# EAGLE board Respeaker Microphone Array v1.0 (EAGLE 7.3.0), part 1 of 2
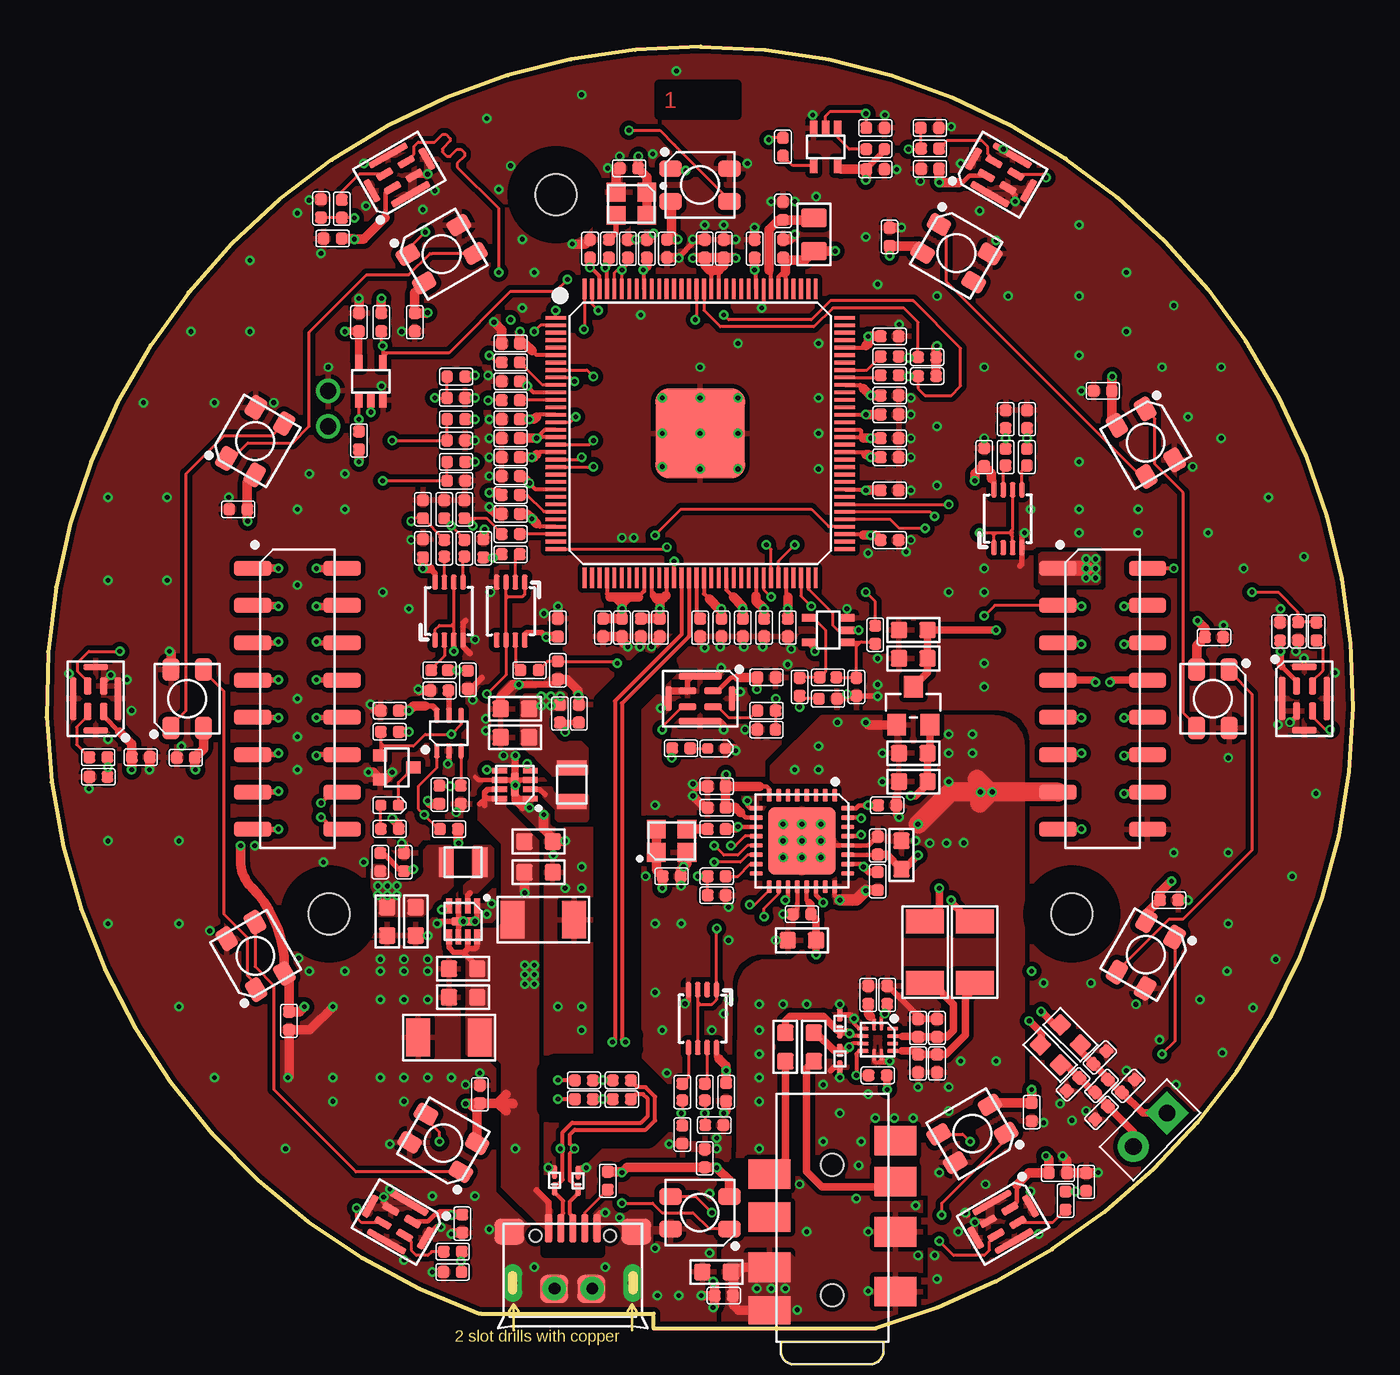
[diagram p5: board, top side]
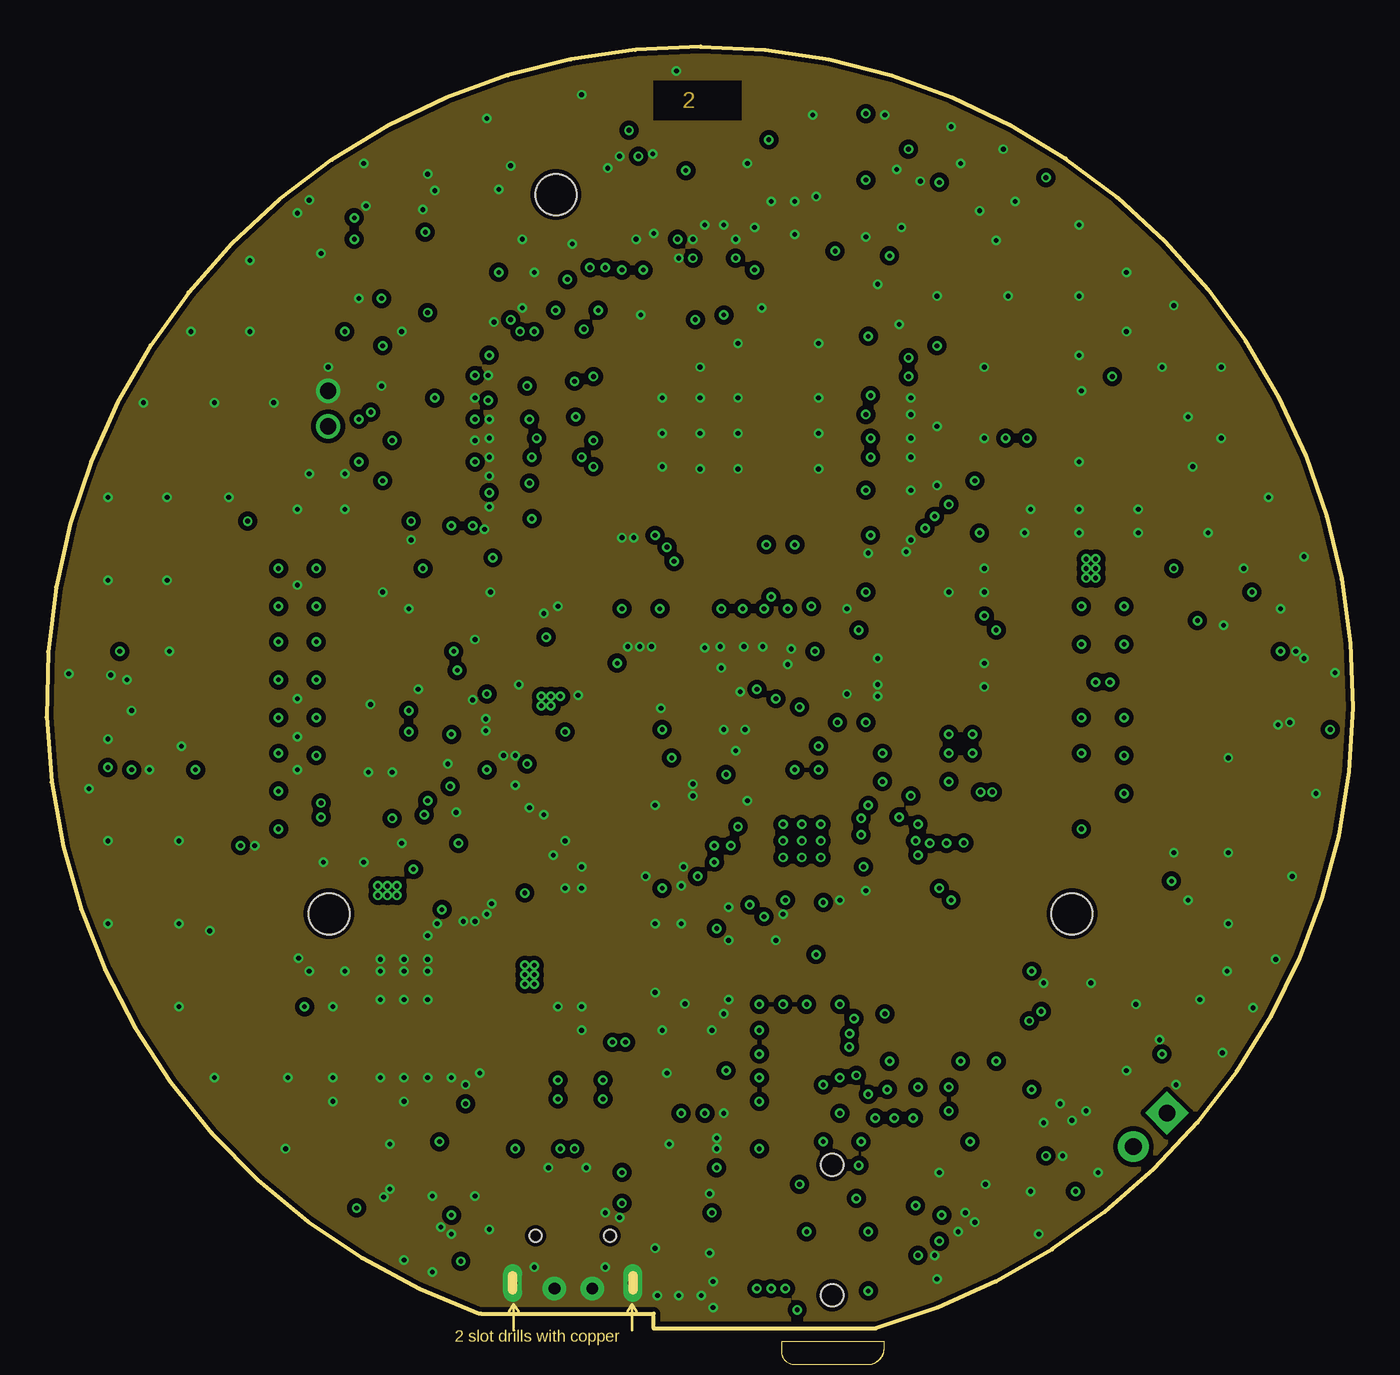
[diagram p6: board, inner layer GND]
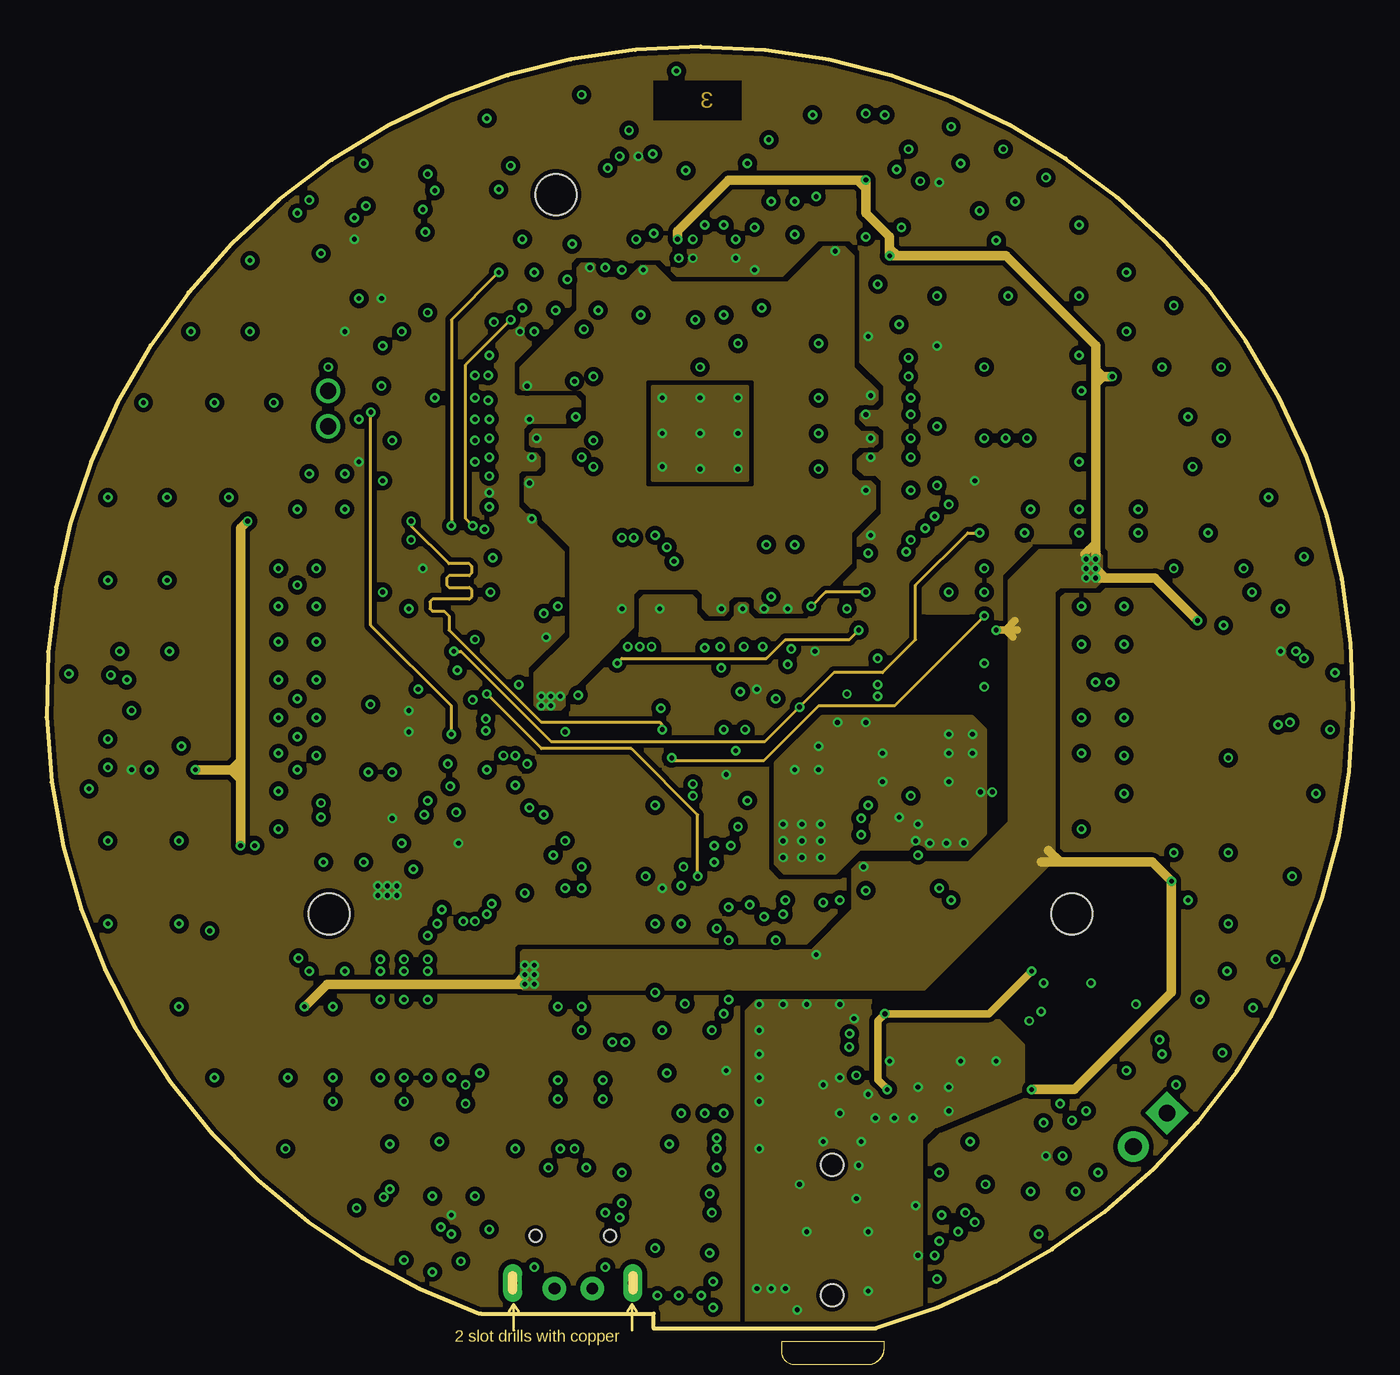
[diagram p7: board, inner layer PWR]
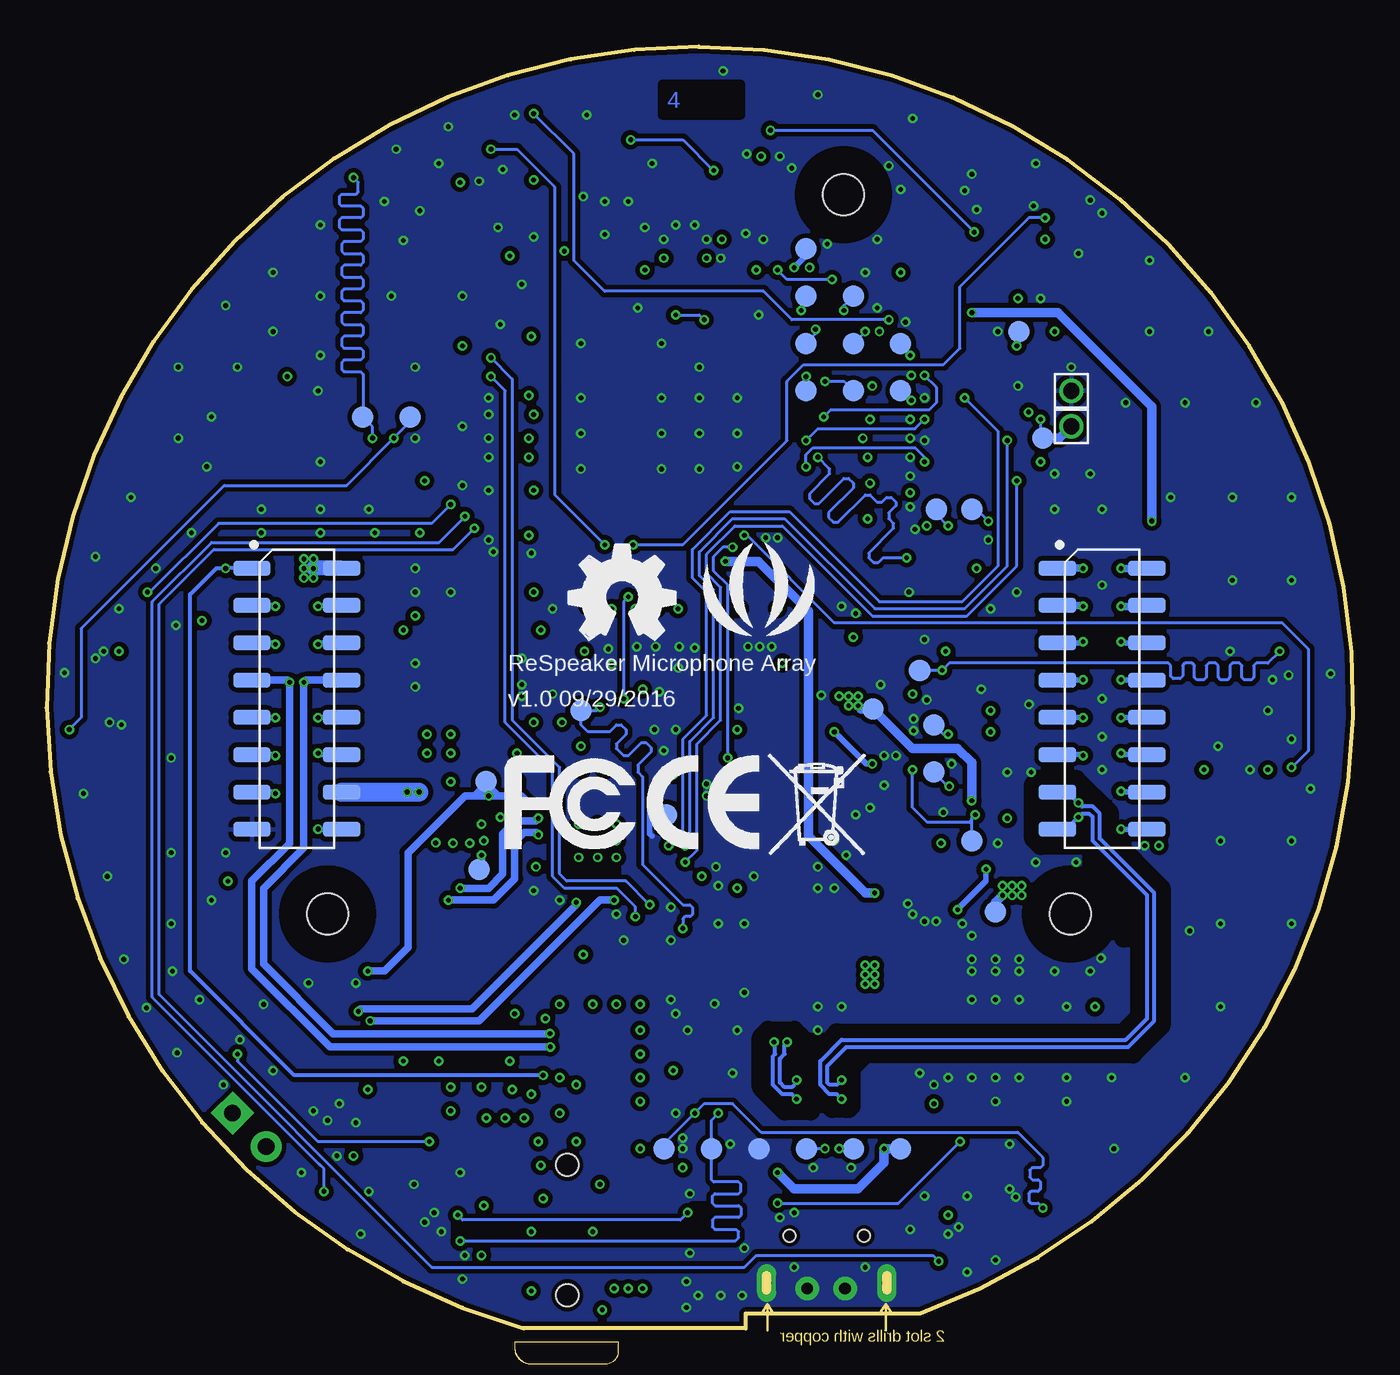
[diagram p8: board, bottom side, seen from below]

Size 70.04 x 68.72 mm. Coordinates in mm from the lower left corner, seen from the top.
Outline: 32.55,0 44.46,0
Outline: 23.28,0.79 32.55,0.79 32.55,0.03
Outline: 35.06,68.72 arc-164 44.47,0.01
Outline: 35.06,68.71 arc161 23.23,0.79
Copper layers (1*2*15*16): Top 0.035mm / dielectric 0.2mm / GND 0.0175mm / dielectric 0.3mm / PWR 0.0175mm / dielectric 0.2mm / Bottom 0.035mm
Design rules "SeeedStudio_4layer_DRU_no_angle_20140221 *": minimum track width 1mil, minimum drill 8mil, track to track 6mil, track to pad 6mil, pad to pad 6mil, via to via 6mil, smd to smd 0mil, copper to edge 10mil, drill to drill 8mil, minimum pad ring 6mil, minimum via ring 4mil, stop-mask expansion 4mil, vias tented up to drill 25mil, thermal gap 10mil
Net classes: 0 default: width 0.025 mm, drill 0.203 mm, clearance 0.102 mm
Holes 2.2 mm at 15.14,22.22 54.98,22.22 27.3,60.78
tRestrict: area 22.1,24.2 to 22.5,25.8; area 27.4,28.9 to 28.9,29.4; area 52.6,19.9 to 57.3,24.6; area 12.8,19.9 to 17.5,24.6; area 25,58.4 to 29.7,63.1; area 32.8,65 to 37,66.7; area 36.8,8.2 to 37.3,8.9; area 48.2,10.2 to 50.3,11.9; area 34.9,25.2 to 35.4,25.8; 19 lines
bRestrict: area 52.6,19.9 to 57.3,24.6; area 12.8,19.9 to 17.5,24.6; area 25,58.4 to 29.7,63.1; area 32.8,65 to 37,66.7; area 39.5,24.2 to 41.8,24.9; area 35.5,5.1 to 48.1,5.6; area 34.7,6.1 to 35.4,6.6; 33 lines

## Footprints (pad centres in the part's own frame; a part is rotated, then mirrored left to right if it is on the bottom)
TP-D45MIL = smd 1.143 x 1.143: T 0,0
C0402 = smd 0.635 x 0.635: 1 0,0.484; 2 0,-0.484
C0603 = smd 0.889 x 0.889: 1 0,0.762; 2 0,-0.762
C1206 = smd 1.27 x 2.032: 1 -1.651,0; 2 1.651,0
SOD-923 = smd 0.7 x 0.3: 1 -0.45,0; 2 0.45,0
LED-0402 = smd 0.58 x 0.58: + -0.468,0; - 0.468,0
MICRO-USB5+4P-SMD-0.65-B = smd 0.381 x 1.524: 1 -1.3,-0.25; 2 -0.65,-0.25; 3 0,-0.25; 4 0.65,-0.25; 5 1.3,-0.25 | smd 1.6 x 1.397: S1 -3.4,-0.427; S6 3.4,-0.427 | drill 0.508 pad 1.016 long: S2 -3.226,-3.175; S5 3.226,-3.175 | smd 1.5 x 1.5: S3 -1,-3.5; S4 1,-3.5 | hole 0.635: -2,-0.65; 2,-0.65
H2X8-SMD-2.0 = smd 2 x 0.8: 1 -2.4,7; 2 2.4,7; 3 -2.4,5; 4 2.4,5; 5 -2.4,3; 6 2.4,3; 7 -2.4,1; 8 2.4,1; 9 -2.4,-1; 10 2.4,-1; 11 -2.4,-3; 12 2.4,-3; 13 -2.4,-5; 14 2.4,-5; 15 -2.4,-7; 16 2.4,-7
1P-40/25MIL = drill 0.864 pad 1.27: 1 0,0
AUDIO8P-SMD-3.5-14.5X6.1X4.0MM = smd 1.6 x 2.25: 1 3.9,-3.375; 2 7.1,-3.375; 3 9.8,-3.375; 4 10.2,3.375; 6 5.2,3.375; 7 7.9,3.375; 8 12,-3.375 | smd 1.5 x 2.25: 5 2.9,3.375 | hole 1.2: 3.7,0; 10.7,0
H2-2.54 = drill 0.889 pad 1.651 square: 1 0,1.27 | drill 0.889 pad 1.651: 2 0,-1.27
L201610 = smd 0.8 x 1.6: 1 -0.9,0; 2 0.9,0
L0603 = smd 0.889 x 0.889: 1 -0.762,0; 2 0.762,0
HCLGA5P-3X4X1MM = smd 0.95 x 0.4: 1 -0.675,-0.425; 2 0.675,-0.425; 3 0.675,0.425; 4 -0.675,0.425 | smd 2.3 x 0.35: 5 0,-1.2; 7 0,1.2 | smd 0.35 x 1.3: 6 1.7,0; 8 -1.7,0
SOT-323 = smd 0.635 x 0.762: 1 -0.635,-0.889; 2 0.635,-0.889; 3 0,0.889
R0402 = smd 0.635 x 0.635: 1 0,0.484; 2 0,-0.484
R0805 = smd 1.397 x 1.016: 1 0,0.889; 2 0,-0.889
R0402' = smd 0.635 x 0.635: 1 0,0.445; 2 0,-0.445
LED4-SMD-3.5X3.7MM = smd 1.2 x 0.9: 1 -1.58,0.875; 2 -1.58,-0.875; 3 1.58,-0.875; 4 1.58,0.875
LEAD12P-SMD-0.4-1.8X1.8X0.5MM = smd 0.6 x 0.2: 1 -0.8,0.2; 2 -0.8,-0.2; 7 0.8,-0.2; 8 0.8,0.2 | smd 0.2 x 0.6: 3 -0.6,-0.8; 4 -0.2,-0.8; 5 0.2,-0.8; 6 0.6,-0.8; 9 0.6,0.8; 10 0.2,0.8; 11 -0.2,0.8; 12 -0.6,0.8
TQFP128-0.4-14X14MM = smd 1.1 x 0.2: 1 -7.75,6.2; 2 -7.75,5.8; 3 -7.75,5.4; 4 -7.75,5; 5 -7.75,4.6; 6 -7.75,4.2; 7 -7.75,3.8; 8 -7.75,3.4; 9 -7.75,3; 10 -7.75,2.6; 11 -7.75,2.2; 12 -7.75,1.8; 13 -7.75,1.4; 14 -7.75,1; 15 -7.75,0.6; 16 -7.75,0.2; 17 -7.75,-0.2; 18 -7.75,-0.6; 19 -7.75,-1; 20 -7.75,-1.4; 21 -7.75,-1.8; 22 -7.75,-2.2; 23 -7.75,-2.6; 24 -7.75,-3; 25 -7.75,-3.4; 26 -7.75,-3.8; 27 -7.75,-4.2; 28 -7.75,-4.6; 29 -7.75,-5; 30 -7.75,-5.4; 31 -7.75,-5.8; 32 -7.75,-6.2; 65 7.75,-6.2; 66 7.75,-5.8; 67 7.75,-5.4; 68 7.75,-5; 69 7.75,-4.6; 70 7.75,-4.2; 71 7.75,-3.8; 72 7.75,-3.4; 73 7.75,-3; 74 7.75,-2.6; 75 7.75,-2.2; 76 7.75,-1.8; 77 7.75,-1.4; 78 7.75,-1; 79 7.75,-0.6; 80 7.75,-0.2; 81 7.75,0.2; 82 7.75,0.6; 83 7.75,1; 84 7.75,1.4; 85 7.75,1.8; 86 7.75,2.2; 87 7.75,2.6; 88 7.75,3; 89 7.75,3.4; 90 7.75,3.8; 91 7.75,4.2; 92 7.75,4.6; 93 7.75,5; 94 7.75,5.4; 95 7.75,5.8; 96 7.75,6.2 | smd 0.2 x 1.1: 33 -6.2,-7.75; 34 -5.8,-7.75; 35 -5.4,-7.75; 36 -5,-7.75; 37 -4.6,-7.75; 38 -4.2,-7.75; 39 -3.8,-7.75; 40 -3.4,-7.75; 41 -3,-7.75; 42 -2.6,-7.75; 43 -2.2,-7.75; 44 -1.8,-7.75; 45 -1.4,-7.75; 46 -1,-7.75; 47 -0.6,-7.75; 48 -0.2,-7.75; 49 0.2,-7.75; 50 0.6,-7.75; 51 1,-7.75; 52 1.4,-7.75; 53 1.8,-7.75; 54 2.2,-7.75; 55 2.6,-7.75; 56 3,-7.75; 57 3.4,-7.75; 58 3.8,-7.75; 59 4.2,-7.75; 60 4.6,-7.75; 61 5,-7.75; 62 5.4,-7.75; 63 5.8,-7.75; 64 6.2,-7.75; 97 6.2,7.75; 98 5.8,7.75; 99 5.4,7.75; 100 5,7.75; 101 4.6,7.75; 102 4.2,7.75; 103 3.8,7.75; 104 3.4,7.75; 105 3,7.75; 106 2.6,7.75; 107 2.2,7.75; 108 1.8,7.75; 109 1.4,7.75; 110 1,7.75; 111 0.6,7.75; 112 0.2,7.75; 113 -0.2,7.75; 114 -0.6,7.75; 115 -1,7.75; 116 -1.4,7.75; 117 -1.8,7.75; 118 -2.2,7.75; 119 -2.6,7.75; 120 -3,7.75; 121 -3.4,7.75; 122 -3.8,7.75; 123 -4.2,7.75; 124 -4.6,7.75; 125 -5,7.75; 126 -5.4,7.75; 127 -5.8,7.75; 128 -6.2,7.75 | smd 4.8 x 4.8: PAD 0,0
DFN8G-0.5-2X2MM = smd 0.8 x 0.3: 1 -0.827,0.75; 2 -0.827,0.25; 3 -0.827,-0.25; 4 -0.827,-0.75; 5 0.827,-0.75; 6 0.827,-0.25; 7 0.827,0.25; 8 0.827,0.75 | smd 0.45 x 1.3: 9 0,0
SOT-353 = smd 0.4 x 0.8: 1 -0.65,-1; 2 0,-1; 3 0.65,-1; 4 0.65,1; 5 -0.65,1
SC-70-6 = smd 0.3 x 0.8: 1 -0.65,-0.95; 2 0,-0.95; 3 0.65,-0.95; 4 0.65,0.95; 5 0,0.95; 6 -0.65,0.95
QFN32G-0.5-5X5MM = smd 0.7 x 0.25: 1 -2.45,1.75; 2 -2.45,1.25; 3 -2.45,0.75; 4 -2.45,0.25; 5 -2.45,-0.25; 6 -2.45,-0.75; 7 -2.45,-1.25; 8 -2.45,-1.75; 17 2.45,-1.75; 18 2.45,-1.25; 19 2.45,-0.75; 20 2.45,-0.25; 21 2.45,0.25; 22 2.45,0.75; 23 2.45,1.25; 24 2.45,1.75 | smd 0.25 x 0.7: 9 -1.75,-2.45; 10 -1.25,-2.45; 11 -0.75,-2.45; 12 -0.25,-2.45; 13 0.25,-2.45; 14 0.75,-2.45; 15 1.25,-2.45; 16 1.75,-2.45; 25 1.75,2.45; 26 1.25,2.45; 27 0.75,2.45; 28 0.25,2.45; 29 -0.25,2.45; 30 -0.75,2.45; 31 -1.25,2.45; 32 -1.75,2.45 | smd 3.6 x 3.6: 33 0,0
SOT-23 = smd 1.016 x 1.143: 1 -0.889,-1.016; 2 0.889,-1.016; 3 0,1.016
US-8 = smd 0.8 x 0.3: 1 -1.55,0.75; 2 -1.55,0.25; 3 -1.55,-0.25; 4 -1.55,-0.75; 5 1.55,-0.75; 6 1.55,-0.25; 7 1.55,0.25; 8 1.55,0.75
OSC-SMD-2.5X2.0X0.9MM = smd 1 x 1: 1 -0.825,-0.625; 2 0.825,-0.625; 3 0.825,0.625; 4 -0.825,0.625

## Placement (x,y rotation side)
1V  [TP-D45MIL]  25.74,33.21 90 bottom
3V3  [TP-D45MIL]  19.17,22.34 180 bottom
24M  [TP-D45MIL]  29.33,57.89 270 bottom
24M_1  [TP-D45MIL]  36.81,27.53 0 bottom
ADM_VIN  [TP-D45MIL]  22.46,29.82 270 bottom
C1  100nF  [C0402]  36.43,12.67 180 top
C2  100nF  [C0402]  33.51,24.23 270 top
C3  10uF  [C0603]  46.47,37.44 90 top
C4  100nF  [C0402]  44.56,25.88 0 top
C5  100nF  [C0402]  27.41,37.57 0 top
C6  10uF  [C0603]  22.33,19.28 90 top
C7  10uF  [C0603]  22.33,17.75 90 top
C8  10uF  [C0603]  18.27,21.82 180 top
C9  10uF  [C0603]  19.79,21.82 180 top
C10  100uF 10V  [C1206]  21.57,15.6 0 top
C11  100nF  [C0402]  19.73,53.95 180 top
C12  100nF  [C0402]  10.27,43.91 90 top
C13  100nF  [C0402]  7.46,30.6 90 top
C14  100nF  [C0402]  13,16.49 180 top
C15  100nF  [C0402]  23.23,12.55 0 top
C16  100nF  [C0402]  35.29,9.12 0 top
C17  10uF  [C0603]  46.47,35.92 90 top
C18  10uF  [C0603]  25.11,31.69 90 top
C19  10uF  [C0603]  26.38,26.1 270 top
C20  10uF  [C0603]  25.11,33.21 90 top
C21  10uF  [C0603]  26.38,24.45 270 top
C22  100uF 10V  [C1206]  26.63,21.91 180 top
C23  100nF  [C0402]  39.48,59.91 0 top
C24  100nF  [C0402]  31.23,62.2 90 top
C25  100nF  [C0402]  45.2,44.93 270 top
C26  100nF  [C0402]  32.18,57.89 0 top
C27  100nF  [C0402]  45.2,50.01 270 top
C28  100nF  [C0402]  24.88,47.73 90 top
C29  100nF  [C0402]  24.88,50.77 90 top
C30  100nF  [C0402]  45.2,47.73 270 top
C31  100nF  [C0402]  39.49,57.89 0 top
C32  100nF  [C0402]  29.14,57.89 0 top
C33  100nF  [C0402]  24.88,45.69 90 top
C34  100nF  [C0402]  29.83,37.57 180 top
C35  100nF  [C0402]  30.85,37.57 180 top
C36  100nF  [C0402]  36.18,37.57 180 top
C37  100nF  [C0402]  38.47,37.57 180 top
C38  100nF  [C0402]  39.74,37.57 180 top
C39  100nF  [C0402]  35.3,57.89 0 top
C40  100nF  [C0402]  24.88,43.66 90 top
C41  100nF  [C0402]  32.88,37.57 180 top
C42  100nF  [C0402]  31.87,37.57 180 top
C43  100nF  [C0402]  24.88,46.71 90 top
C44  100nF  [C0402]  24.88,48.74 90 top
C45  100nF  [C0402]  24.88,52.81 90 top
C46  100nF  [C0402]  37.33,37.57 180 top
C47  100nF  [C0402]  45.2,42.27 270 top
C48  100nF  [C0402]  45.2,46.71 270 top
C49  100nF  [C0402]  45.2,49 270 top
C50  100nF  [C0402]  45.2,53.19 270 top
C51  100nF  [C0402]  37.96,57.89 0 top
C52  100nF  [C0402]  36.31,57.89 0 top
C53  100nF  [C0402]  52.82,11.6 180 top
C54  100nF  [C0402]  60.18,22.97 270 top
C55  100nF  [C0402]  38.6,34.9 270 top
C56  100nF  [C0402]  15.33,58.43 90 top
C57  100nF  [C0402]  5.05,30.63 270 top
C58  100nF  [C0402]  22.28,5.62 180 top
C59  100nF  [C0402]  54.22,8.33 270 top
C60  100nF  [C0402]  66.13,37.36 0 top
C61  100nF  [C0402]  47.37,62.17 90 top
C62  100nF  [C0402]  44.56,23.98 180 top
C63  2.2nF  [C0402]  21.06,34.2 90 top
C64  100nF  [C0402]  18.4,33.12 90 top
C65  100nF  [C0402]  16.74,53.95 0 top
C66  100nF  [C0402]  31.17,57.89 0 top
C67  100nF  [C0402]  50.27,46.71 0 top
C68  10uF  [C0603]  46.47,30.84 90 top
C69  100nF  [C0402]  40.5,22.2 90 top
C70  100nF  [C0402]  20.18,41.82 0 top
C71  10uF  [C0603]  46.47,29.31 90 top
C72  100nF  [C0402]  62.59,37.06 270 top
C73  100nF  [C0402]  56.63,50.26 90 top
C74  100nF  [C0402]  45.19,58.52 0 top
C75  100nF  [C0402]  33.26,57.89 180 top
C76  100nF  [C0402]  44.43,62.14 270 top
C77  1.5nF  [C0402]  22.4,43.92 180 top
C78  100pF  [C0402]  35.92,23.22 270 top
C79  100nF  [C0402]  45.07,17.88 0 top
C80  1.5nF  [C0402]  21.95,45.44 90 top
C81  100nF  [C0402]  44.05,17.88 0 top
C82  1.5nF  [C0402]  21.95,47.6 90 top
C83  1.5nF  [C0402]  21.95,49.89 90 top
C84  100pF  [C0402]  23.42,41.82 0 top
C85  100pF  [C0402]  27.42,35.28 180 top
C86  470pF  [C0402]  41.89,33.76 270 top
C87  470pF  [C0402]  22.59,34.77 180 top
C88  100nF  [C0402]  35.92,29.06 90 top
C89  100nF  [C0402]  45.07,28.04 270 top
C90  100uF 10V  [C1206]  49.77,20.17 270 top
C91  100uF 10V  [C1206]  47.1,20.17 270 top
C92  100pF  [C0402]  46.72,16.1 0 top
C93  100pF  [C0402]  46.72,14.2 180 top
C94  470pF  [C0402]  21.32,43.92 0 top
C95  100pF  [C0402]  55.03,13.08 135 top
C96  100pF  [C0402]  56.47,14.52 315 top
C97  680nF DNP  [C0402]  56.56,12.99 315 top
C98  100pF  [C0402]  56.56,11.56 135 top
C99  100pF  [C0402]  58,12.99 315 top
C100  10uF  [C0603]  40.5,20.8 270 top
C101  470pF  [C0402]  20.18,43.92 0 top
C102  10uF  [C0603]  45.83,25.37 180 top
C103  470pF  [C0402]  34.08,10.39 180 top
C104  470pF  [C0402]  35.8,10.9 270 top
C105  470pF  [C0402]  52.56,48.74 0 top
C106  470pF  [C0402]  51.42,48.74 0 top
C107  100nF  [C0402]  35.92,27.91 90 top
C108  470pF  [C0402]  43.42,34.39 180 top
C109  DNP 330pF  [C0402]  67.1,37.38 180 top
C110  DNP 330pF  [C0402]  55.74,7.85 0 top
C111  DNP 330pF  [C0402]  21.76,3.02 90 top
C112  DNP 330pF  [C0402]  2.78,29.57 90 top
C113  DNP 330pF  [C0402]  38.59,32.11 90 top
C114  DNP 330pF  [C0402]  14.72,60.05 0 top
C115  DNP 330pF  [C0402]  47.35,64.36 270 top
D1  DF2S6.8FS  [SOD-923]  42.53,16.36 90 top
D2  DF2S6.8FS  [SOD-923]  42.53,14.45 270 top
D7  TOSHIBA;DF2S6.8FS(TL4,D)  [SOD-923]  27.23,7.92 90 top
D8  TOSHIBA;DF2S6.8FS(TL4,D)  [SOD-923]  28.49,7.9 90 top
D9  LED_RED  [LED-0402]  35.92,31.09 0 top
D11  LED_GREEN  [LED-0402]  18.4,28.04 0 top
DM  [TP-D45MIL]  26.77,9.63 270 bottom
DP  [TP-D45MIL]  29.31,9.63 270 bottom
FR1  [SEEEDSTUDIO-PCB-FRAME]  not placed on the board
FR2  [SEEEDSTUDIO-PCB-FRAME]  not placed on the board
FR3  [SEEEDSTUDIO-PCB-FRAME]  not placed on the board
FR4  [SEEEDSTUDIO-PCB-FRAME]  not placed on the board
FR5  [SEEEDSTUDIO-PCB-FRAME]  not placed on the board
FR7  [SEEEDSTUDIO-PCB-FRAME]  not placed on the board
FR8  [SEEEDSTUDIO-PCB-FRAME]  not placed on the board
GND  [TP-D45MIL]  31.85,9.63 270 bottom
GND1  [TP-D45MIL]  24.25,9.63 0 bottom
J1  DNP 320010000  [MICRO-USB5+4P-SMD-0.65-B]  28.21,5.61 0 top
J2  320030443  [H2X8-SMD-2.0]  13.45,33.76 0 bottom
J3  320030443  [H2X8-SMD-2.0]  56.63,33.76 0 bottom
J4  [1P-40/25MIL]  15.1,50.27 0 bottom
J5  320030443  [H2X8-SMD-2.0]  13.45,33.76 0 top
J6  320030443  [H2X8-SMD-2.0]  56.63,33.76 0 top
J7  [1P-40/25MIL]  15.1,48.36 0 bottom
J9  DNP AUDIO-JACK-8P-SMD  [AUDIO8P-SMD-3.5-14.5X6.1X4.0MM]  42.12,-1.93 90 top
J10  DNP  [H2-2.54]  59.17,10.64 315 top
L1  0.47uH  [L201610]  22.33,24.99 180 top
L2  0.47uH  [L201610]  28.15,29.15 90 top
L3  BLM18BD252SN1  [L0603]  41.13,15.09 270 top
L4  BLM18BD252SN1  [L0603]  39.61,15.09 270 top
L5  DNP  [L0603]  35.92,3.02 0 top
L6  BLM18BD252SN1  [L0603]  54.89,15.74 315 top
L7  BLM18BD252SN1  [L0603]  53.81,14.66 315 top
MIC7  MP34DT01  [HCLGA5P-3X4X1MM]  35.04,33.76 180 top
MIC8  MP34DT01  [HCLGA5P-3X4X1MM]  18.91,61.85 30 top
MIC9  MP34DT01  [HCLGA5P-3X4X1MM]  2.63,33.76 90 top
MIC10  MP34DT01  [HCLGA5P-3X4X1MM]  18.83,5.69 150 top
MIC11  MP34DT01  [HCLGA5P-3X4X1MM]  51.28,5.71 210 top
MIC12  MP34DT01  [HCLGA5P-3X4X1MM]  67.44,33.77 270 top
MIC13  MP34DT01  [HCLGA5P-3X4X1MM]  51.17,61.85 330 top
MIC_CLK0  [TP-D45MIL]  20.43,43.91 270 bottom
MIC_CLK1  [TP-D45MIL]  22.34,43.91 270 bottom
MIC_CLK2  [TP-D45MIL]  23.23,35.28 270 bottom
MIC_CLK3  [TP-D45MIL]  36.94,9.62 270 bottom
MIC_CLK4  [TP-D45MIL]  34.4,9.62 270 bottom
MIC_CLK5  [TP-D45MIL]  50.54,48.86 90 bottom
MIC_CLK6  [TP-D45MIL]  53.08,48.86 90 bottom
PG  [TP-D45MIL]  20.43,26.13 180 bottom
PMCK  [TP-D45MIL]  41.39,33.12 180 bottom
POR  [TP-D45MIL]  22.47,32.36 270 bottom
Q1  CJ2102  [SOT-323]  18.78,30.07 270 top
R1  33R  [R0402]  30.15,57.89 0 top
R2  10K  [R0402]  16.75,47.6 0 top
R3  10k  [R0402]  47.74,16.1 0 top
R4  0R  [R0402]  30.84,13.3 90 top
R5  100K_1%  [R0402]  17.89,24.99 0 top
R6  43.2R  [R0402]  35.04,37.57 180 top
R7  22K_1%  [R0402]  19.16,24.99 0 top
R8  0R  [R0402]  28.81,13.3 90 top
R9  0R  [R0402]  28.81,12.28 90 top
R10  20K_1%  [R0402]  27.52,32.96 180 top
R11  30K_1%  [R0402]  28.54,32.96 0 top
R12  33R  [R0402]  24.88,51.79 270 top
R13  4.7R  [R0805]  41.14,58.65 0 top
R14  33R  [R0402]  24.88,49.76 270 top
R15  10k  [R0402]  47.21,52.07 90 top
R16  10k  [R0402]  47.21,51.06 90 top
R17  1k  [R0402]  24.88,44.68 270 top
R18  33R  [R0402]  35.92,24.23 270 top
R19  33R  [R0402]  35.92,26.77 90 top
R20  100k  [R0402]  44.56,13.56 270 top
R21  10K  [R0402]  21.57,26.77 90 top
R22  10K  [R0402]  22.21,28.61 180 top
R23  3.9k  [R0402]  21.06,28.61 0 top
R24  10K  [R0402]  18.4,31.98 90 top
R25  470R  [R0402]  18.4,26.78 90 top
R26  33R  [R0402']  22.4,41.82 180 top
R27  10K  [R0402]  17.94,53.95 180 top
R28  33R  [R0402']  21.06,35.28 90 top
R29  33R  [R0402']  21.32,41.82 180 top
R30  33R  [R0402']  35.29,12.67 0 top
R31  33R  [R0402']  34.08,12.67 0 top
R32  0R  [R0402]  36.31,1.75 90 top
R33  33R  [R0402]  21.95,51.03 90 top
R34  470R  [R0402]  34.02,31.09 270 top
R35  10K  [R0402]  44.43,63.22 90 top
R36  0R DNP  [R0402]  45.2,51.09 270 top
R37  0R DNP  [R0402]  45.2,52.11 270 top
R38  0R  [R0402]  30.84,12.28 90 top
R39  10k  [R0402]  47.74,14.2 180 top
R40  33R  [R0402]  21.95,48.74 90 top
R41  33R  [R0402]  21.95,46.46 90 top
R42  DNP 0R  [R0402']  41.9,34.9 270 top
R43  DNP 10K  [R0402]  30.08,7.92 0 top
R44  33R  [R0402]  39.48,63.35 0 top
R45  10K  [R0402]  44.43,64.36 270 top
R46  33R  [R0402]  40.37,34.39 180 top
R47  33R  [R0402]  24.88,42.59 270 top
R48  33R  [R0402]  44.43,37.19 0 top
R49  33R  [R0402]  24.88,41.5 90 top
R50  33R  [R0402]  25.89,35.29 270 top
R52  33R  [R0402']  51.41,46.71 180 top
R53  33R  [R0402']  52.56,46.71 180 top
R58  33R  [R0402]  68.08,37.37 180 top
R60  33R  [R0402]  54.63,6.85 180 top
R61  33R  [R0402]  21.77,4.11 90 top
R62  33R  [R0402]  2.77,30.61 90 top
R63  33R  [R0402]  47.37,63.25 90 top
R64  33R  [R0402]  15.82,60.03 180 top
R65  33R  [R0402]  38.6,33.12 270 top
RST  [TP-D45MIL]  17.9,53.44 0 bottom
RST_N  [TP-D45MIL]  16.63,47.73 180 bottom
SK0  SK6812MINI  [LED4-SMD-3.5X3.7MM]  35.04,61.3 180 top
SK1  SK6812MINI  [LED4-SMD-3.5X3.7MM]  21.17,57.6 210 top
SK2  SK6812MINI  [LED4-SMD-3.5X3.7MM]  11.18,47.57 240 top
SK3  SK6812MINI  [LED4-SMD-3.5X3.7MM]  7.54,33.76 270 top
SK4  SK6812MINI  [LED4-SMD-3.5X3.7MM]  11.2,19.96 300 top
SK5  SK6812MINI  [LED4-SMD-3.5X3.7MM]  21.27,9.94 330 top
SK6  SK6812MINI  [LED4-SMD-3.5X3.7MM]  35.02,6.2 0 top
SK7  SK6812MINI  [LED4-SMD-3.5X3.7MM]  49.64,10.43 30 top
SK8  SK6812MINI  [LED4-SMD-3.5X3.7MM]  58.93,20.03 60 top
SK9  SK6812MINI  [LED4-SMD-3.5X3.7MM]  62.53,33.76 90 top
SK10  SK6812MINI  [LED4-SMD-3.5X3.7MM]  58.93,47.49 120 top
SK11  SK6812MINI  [LED4-SMD-3.5X3.7MM]  48.78,57.65 150 top
SW1  FSA2275  [LEAD12P-SMD-0.4-1.8X1.8X0.5MM]  44.56,15.47 270 top
TCK  [TP-D45MIL]  29.33,52.81 90 bottom
TDI  [TP-D45MIL]  26.79,52.81 90 bottom
TDO  [TP-D45MIL]  26.79,55.35 90 bottom
TMS  [TP-D45MIL]  29.33,55.35 90 bottom
TP4  [TP-D45MIL]  46.47,29.31 270 bottom
TP14  [TP-D45MIL]  46.85,24.61 180 bottom
U1  XVSM-2000  [TQFP128-0.4-14X14MM]  35.04,47.98 0 top
U2  ETA3410  [DFN8G-0.5-2X2MM]  22.33,21.82 270 top
U3  ETA3410  [DFN8G-0.5-2X2MM]  25.11,29.15 180 top
U4  74HC1G08  [SOT-353]  17.38,50.77 0 top
U5  ADM1085  [SC-70-6]  21.57,31.91 0 top
U6  WM8960  [QFN32G-0.5-5X5MM]  40.5,26.14 270 top
U7  AP7333  [SOT-23]  46.47,33.38 0 top
U8  74AHC1G79  [SOT-353]  41.9,37.44 90 top
U9  NC7NZ34  [US-8]  21.58,38.46 90 top
U10  NC7NZ34  [US-8]  35.16,16.61 270 top
U11  NC7NZ34  [US-8]  51.54,43.41 90 top
U12  NC7NZ34  [US-8]  24.88,38.46 270 top
U13  74HC1G08  [SOT-353]  41.77,63.35 180 top
U$36  [OSHW_FILLX200_NOTEXT_TNAME]  42.02,36.93 0 bottom
U$51  [SEEED-SILK-TNAME-280*268MIL]  31.86,38.84 0 bottom
X1  24MHz  [OSC-SMD-2.5X2.0X0.9MM]  31.35,60.29 180 top
X2  24MHz  [OSC-SMD-2.5X2.0X0.9MM]  33.51,26.14 0 top
XL_DN0  [TP-D45MIL]  26.79,50.27 90 bottom
XL_DN1  [TP-D45MIL]  29.33,50.27 90 bottom
XL_UP0  [TP-D45MIL]  24.25,52.81 90 bottom
XL_UP1  [TP-D45MIL]  24.25,50.27 90 bottom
